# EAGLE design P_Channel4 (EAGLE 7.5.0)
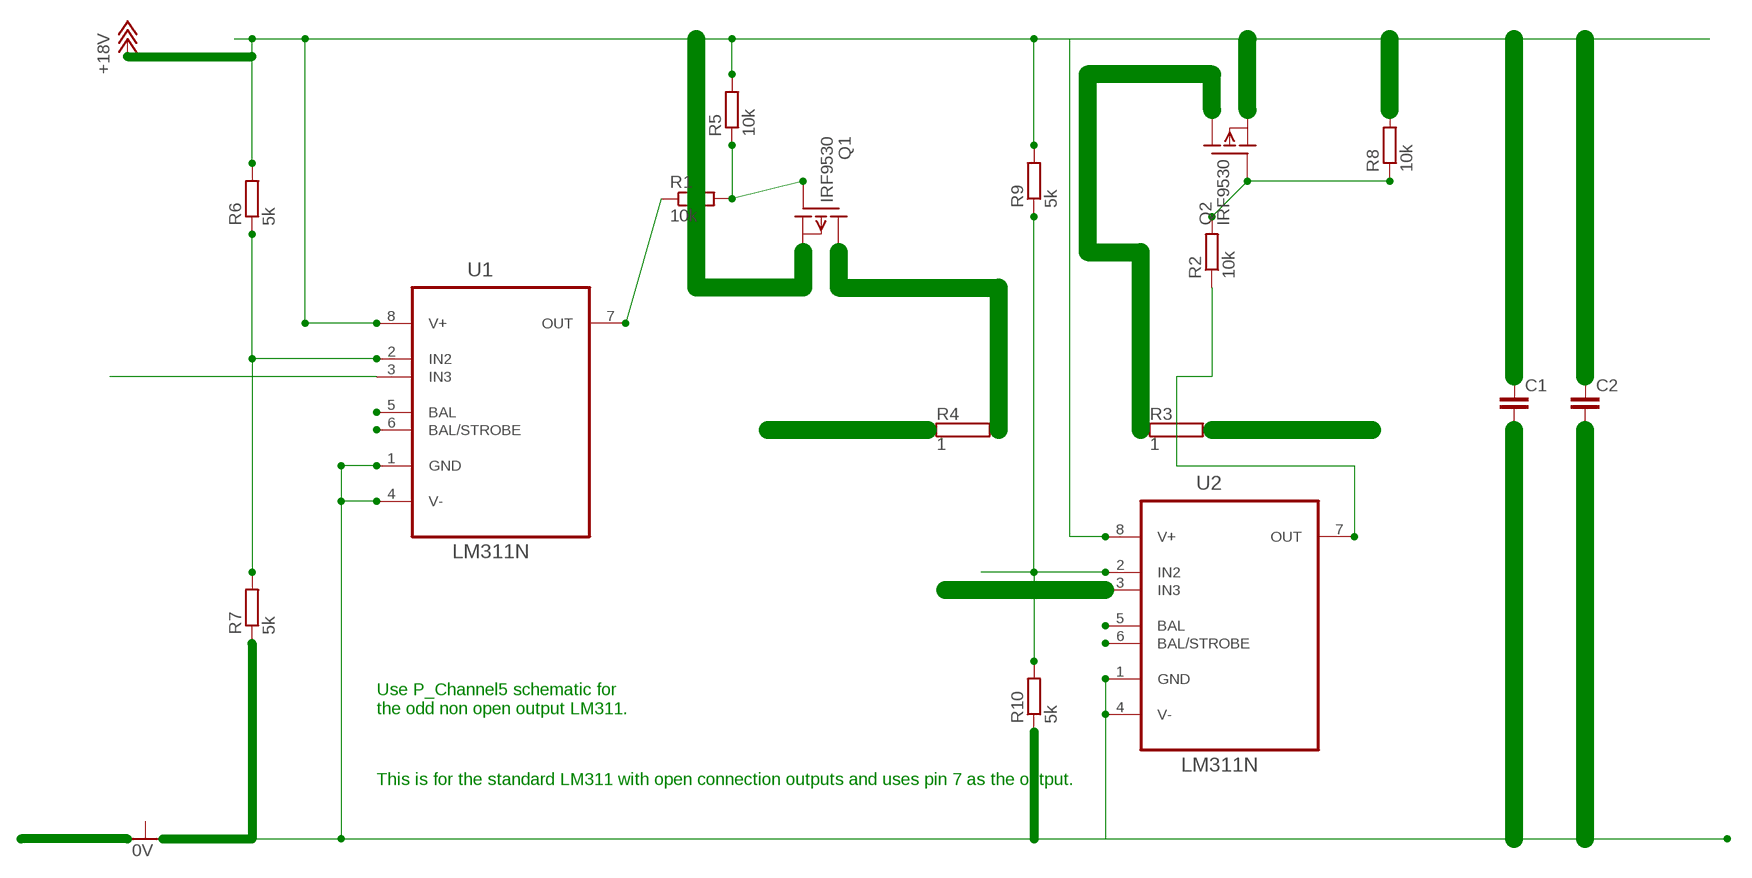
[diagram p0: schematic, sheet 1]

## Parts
C1  C7.5/3  [C7.5B3]
C2  C7.5/3  [C7.5B3]
Q1  IRF9530  [TO220]
Q2  IRF9530  [TO220]
R1  10k  R-EU_0207/10  [0207/10]
R2  10k  R-EU_0207/10  [0207/10]
R3  1  RMG100-H  [TO-247-2H]
R4  1  RMG100-H  [TO-247-2H]
R5  10k  R-EU_0207/10  [0207/10]
R6  5k  R-EU_0207/10  [0207/10]
R7  5k  R-EU_0207/10  [0207/10]
R8  10k  R-EU_0207/10  [0207/10]
R9  5k  R-EU_0207/10  [0207/10]
R10  5k  R-EU_0207/10  [0207/10]
U1  LM311N  [DIP254P762X508-8]
U2  LM311N  [DIP254P762X508-8]

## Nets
+18V: C1.1 C1.2 C2.1 C2.2 Q1.3(S) Q2.3(S) R5.2 R6.2 R7.1 R9.2 R10.1 U1.1(GND) U1.4(V-) U1.8(V+) U2.1(GND) U2.4(V-) U2.8(V+)
N$1: Q1.1(G) R1.2 R5.1
N$2: Q2.1(G) R2.2 R8.1
N$4: Q2.2(D) R3.1
N$5: U1.5(BAL)
N$6: R1.1 U1.7(OUT)
N$7: Q1.2(D) R2.1 R3.2 R4.1 R4.2 U2.3(IN3) U2.7(OUT)
N$8: R6.1 R7.2 R9.1 R10.2 U1.2(IN2) U2.2(IN2)
N$10: U1.3(IN3)
N$11: U1.6(BAL/STROBE)
N$12: U2.5(BAL)
N$13: U2.6(BAL/STROBE)
Unconnected: R8.2

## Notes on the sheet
- Use P_Channel5 schematic for 
  the odd non open output LM311.
- This is for the standard LM311 with open connection outputs and uses pin 7 as the output.

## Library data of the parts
C1 C2 = capacitor-wima:C: CAPACITOR
Q1 Q2 = transistor-fet:IRF9530: P-Channel Enhancement MOSFET (HEXFET); -100V; -12A; 0,3Ohm
R1 R2 R5-R10 = rcl:R-EU_: RESISTOR, European symbol
R3 R4 = resistor-power:RMG100: TO-247 Power Resistor - RMG 100 Series; OC_FARNELL: unknown; OC_NEWARK: unknown
U1 U2 = NSC_By_element14_Batch_1.1:LM311N: Voltage Comparator; MPN: LM311N; OC_FARNELL: 9487220; OC_NEWARK: 07B6414; PACKAGE: DIP-8; SUPPLIER: NationalSemiconductor

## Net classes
0 default: clearance 0.205 mm

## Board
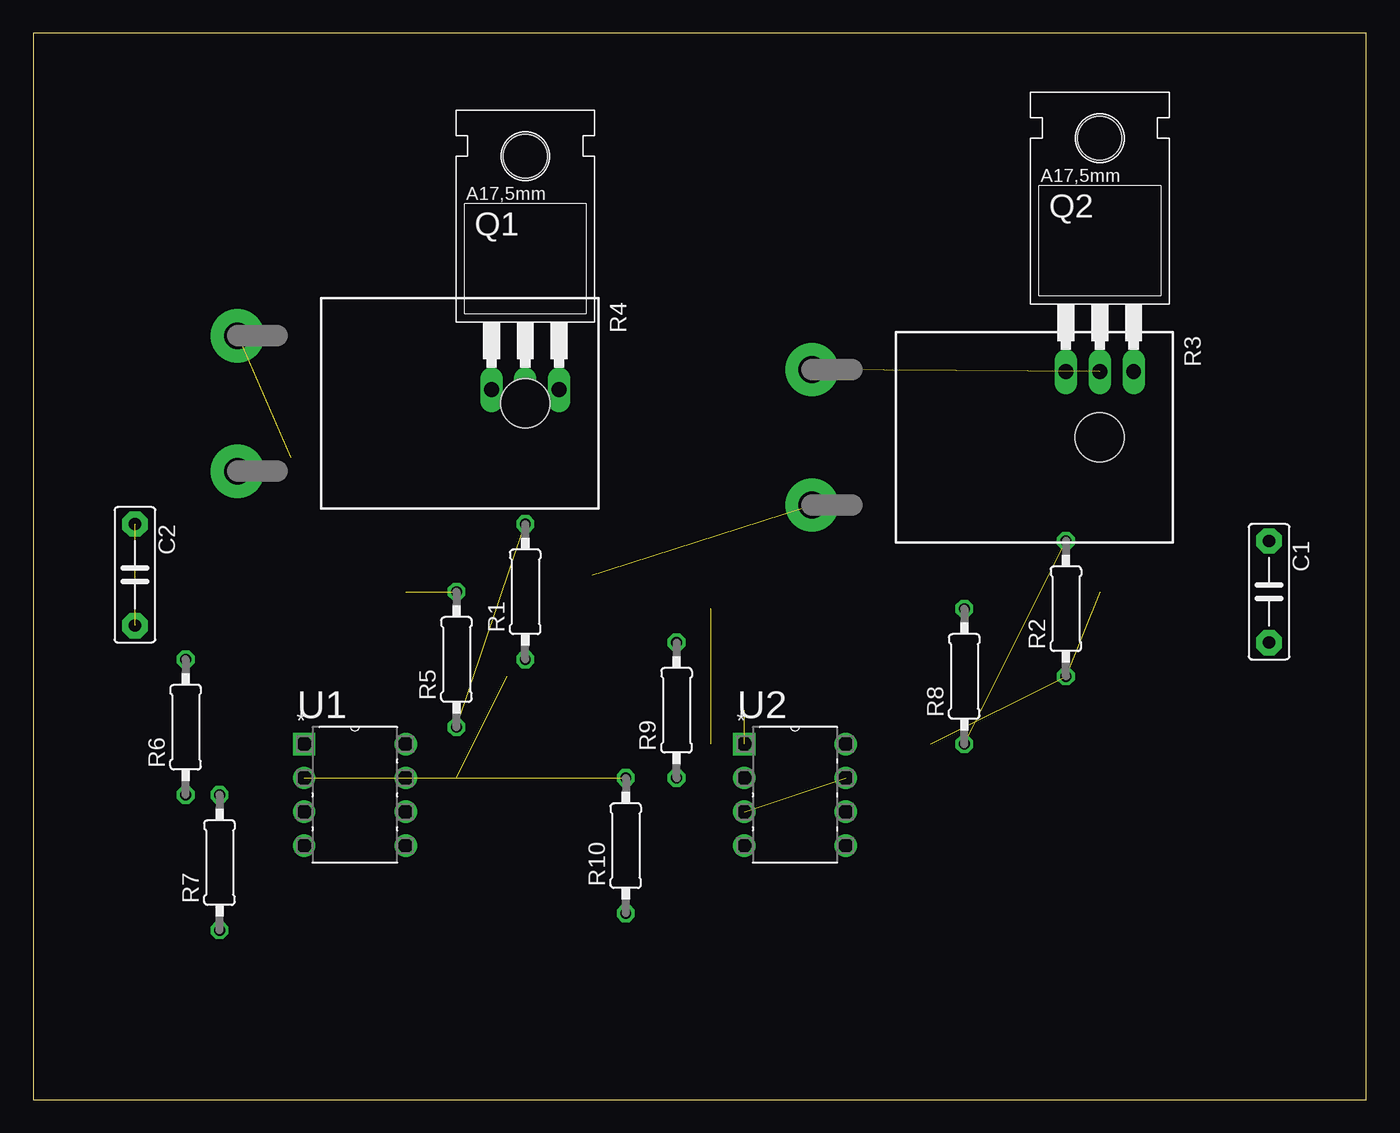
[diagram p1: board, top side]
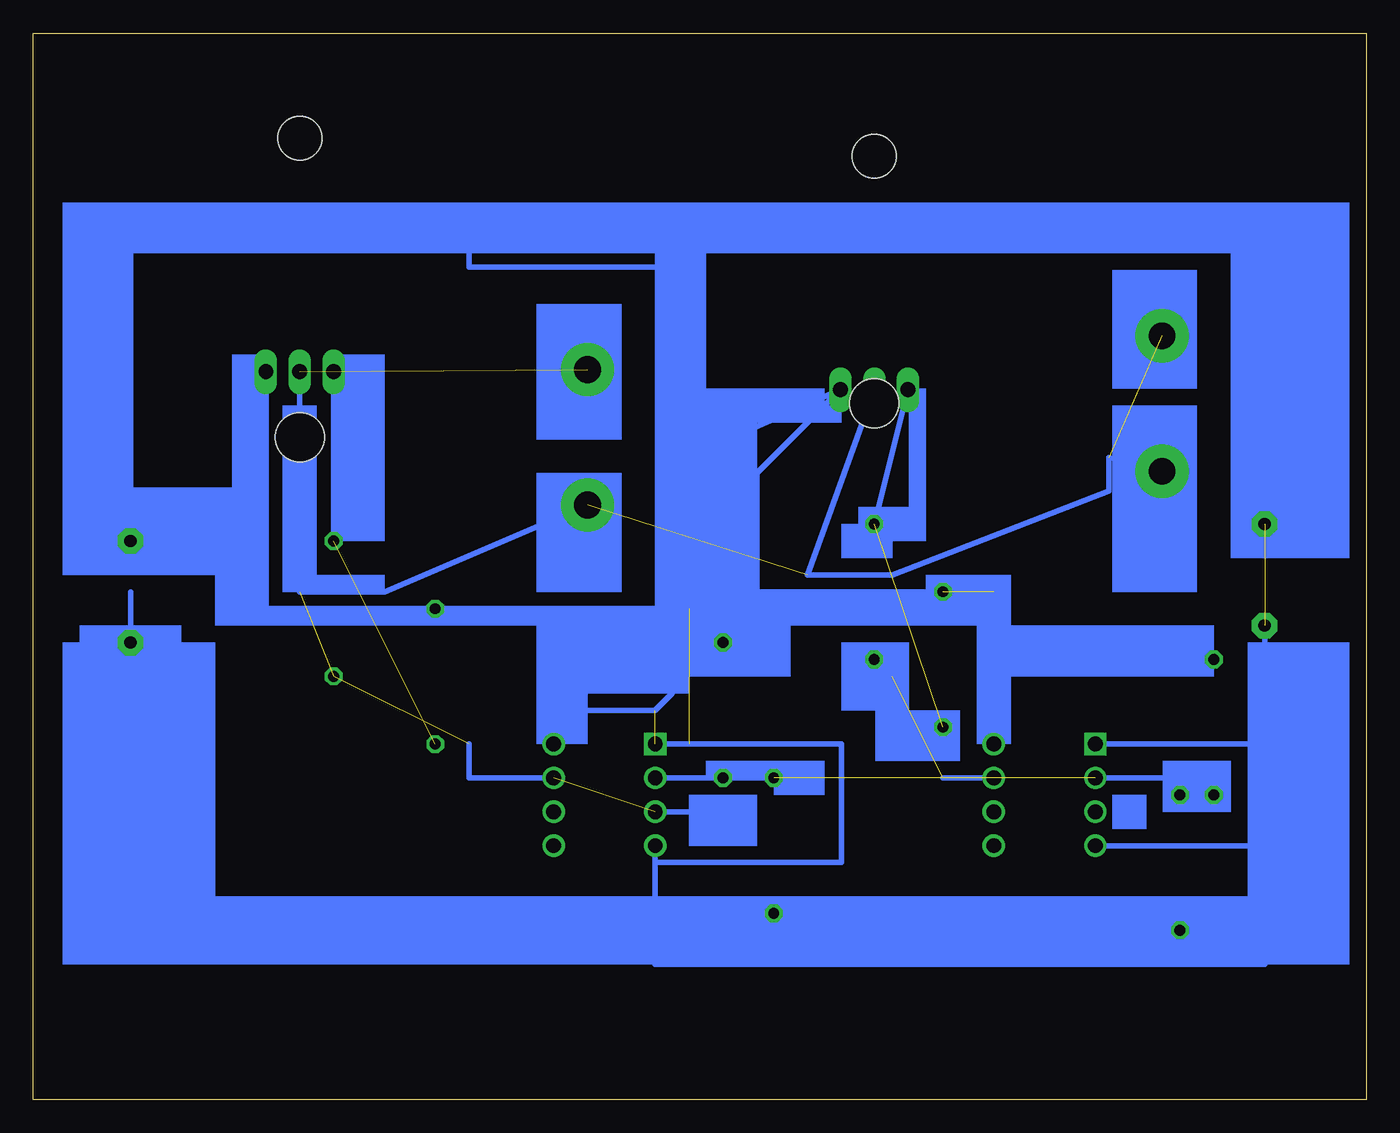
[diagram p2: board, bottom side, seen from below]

Size 100 x 80 mm. Coordinates in mm from the lower left corner, seen from the top.
Outline: 0,0 100,0 100,80 0,80 0,0
Copper layers (1*16): Top 0.035mm / dielectric 1.5mm / Bottom 0.035mm
Design rules "default": minimum track width 10mil, minimum drill 24mil, track to track 8mil, track to pad 8mil, pad to pad 8mil, via to via 8mil, smd to smd 8mil, copper to edge 40mil, drill to drill 8mil, minimum pad ring 10mil, minimum via ring 8mil, stop-mask expansion 4mil, vias tented up to drill 0mil, thermal gap 10mil

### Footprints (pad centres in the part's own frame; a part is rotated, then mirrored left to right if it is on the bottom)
C7.5B3 = drill 0.914 pad 1.905 octagon: 1 -3.81,0; 2 3.81,0
TO220 = drill 1.118 long: 1 -2.54,-6.35; 2 0,-6.35; 3 2.54,-6.35 | hole 3.302: 0,11.176
0207/10 = drill 0.813 octagon: 1 -5.08,0; 2 5.08,0
TO-247-2H = drill 2 pad 4: 1 -5.08,-21.59; 2 5.08,-21.59 | hole 3.7: 0,0
DIP254P762X508-8 = drill 1.118 square: 1 -7.62,7.62 | drill 1.118: 2 -7.62,5.08; 3 -7.62,2.54; 4 -7.62,0; 5 0,0; 6 0,2.54; 7 0,5.08; 8 0,7.62

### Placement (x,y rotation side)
C1  92.71,38.1 270 top
C2  7.62,39.37 270 top
Q1  36.91,59.61 0 top
Q2  80.01,60.96 0 top
R1  36.91,38.1 90 top
R2  77.47,36.83 90 top
R3  80.01,49.69 270 top
R4  36.91,52.23 270 top
R5  31.75,33.02 90 top
R6  11.43,27.94 90 top
R7  13.97,17.78 90 top
R8  69.85,31.75 90 top
R9  48.26,29.21 90 top
R10  44.45,19.05 90 top
U1  27.94,19.05 0 top
U2  60.96,19.05 0 top

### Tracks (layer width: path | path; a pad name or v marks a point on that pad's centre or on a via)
+18V  (4 unrouted)
  Bottom 0.406: 92.71,38.1 C1.2 92.71,12.7 53.34,12.7 | 53.34,12.7 U2.4 53.34,17.78 39.37,17.78 39.37,26.67 U2.1 | C1.1 92.71,45.72 | 92.71,45.72 92.71,63.74 67.31,63.74 67.31,62.47 50.8,62.47 50.8,48.26 | C2.2 7.62,26.67 | 7.62,26.67 U1.1 | 7.62,19.05 7.62,10.16 13.97,10.16 | 13.97,10.16 53.34,10.16 53.34,12.7 | U1.4 7.62,19.05 | 7.62,19.05 7.62,26.67 | R7.1 13.97,10.16 | 27.94,33.02 U1.8 | R6.2 27.94,33.02 | 27.94,33.02 27.94,38.1 45.72,38.1 | 45.72,38.1 45.72,46.99 Q1.3 50.8,48.26 | U2.8 60.96,27.94 59.69,29.21 53.34,29.21 52.07,30.48 52.07,36.83 | 52.07,36.83 82.55,36.83 82.55,45.72 | 82.55,45.72 Q2.3 | 52.07,36.83 50.8,36.83 | 50.8,36.83 R9.2 48.26,35.56 45.72,38.1 | 53.34,12.7 R10.1 | 82.55,45.72 92.71,45.72 | 50.8,48.26 50.8,36.83
N$1  (1 unrouted)
  Bottom 0.406: Q1.1 R1.2
N$2  (1 unrouted)
  Bottom 0.406: R2.2 Q2.1
N$4  (1 unrouted)
N$6  (1 unrouted)
  Bottom 0.406: R1.1 35.56,31.75 | U1.7 31.75,24.13
N$7  (5 unrouted)
  Bottom 0.406: 67.31,26.67 67.31,24.13 U2.7 | U2.3 49.53,21.59 | Q1.2 41.91,39.37 35.56,39.37 19.29,45.64 19.29,48.18 R4.2 | R3.2 73.66,38.1 80.01,38.1 80.01,54.61
N$8  (1 unrouted)
  Bottom 0.406: U1.2 13.97,24.13 R7.2 R6.1 | U2.2 R9.1 R10.2
(copper drawn outside any net)
  shapes: Bottom area x55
